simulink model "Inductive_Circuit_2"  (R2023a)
settings: Solver=VariableStepAuto  StartTime=0.0  StopTime=10.0  RelTol=1e-3
libraries: fl_lib x9

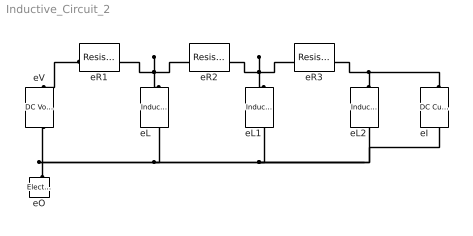
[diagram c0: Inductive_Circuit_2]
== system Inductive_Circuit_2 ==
  eI : fl_lib/Electrical/Electrical Sources/DC Current Source  i0=1 A
  eL : fl_lib/Electrical/Electrical Elements/Inductor  l=1e-6 H  r=0 Ohm  g=1e-9 1/Ohm  i_specify=off  i_priority=None  i=0 A  i_nominal_specify=off  i_nominal_unit=A  i_nominal_value=1  v_specify=off  v_priority=None  v=0 V  v_nominal_specify=off  v_nominal_unit=V  v_nominal_value=1  i_L_specify=off  i_L_priority=High  i_L=0 A  i_L_nominal_specify=off  i_L_nominal_unit=A  i_L_nominal_value=1
  eL1 : fl_lib/Electrical/Electrical Elements/Inductor  l=1e-6 H  r=0 Ohm  g=1e-9 1/Ohm  i_specify=off  i_priority=None  i=0 A  i_nominal_specify=off  i_nominal_unit=A  i_nominal_value=1  v_specify=off  v_priority=None  v=0 V  v_nominal_specify=off  v_nominal_unit=V  v_nominal_value=1  i_L_specify=off  i_L_priority=High  i_L=0 A  i_L_nominal_specify=off  i_L_nominal_unit=A  i_L_nominal_value=1
  eL2 : fl_lib/Electrical/Electrical Elements/Inductor  l=1e-6 H  r=0 Ohm  g=1e-9 1/Ohm  i_specify=off  i_priority=None  i=0 A  i_nominal_specify=off  i_nominal_unit=A  i_nominal_value=1  v_specify=off  v_priority=None  v=0 V  v_nominal_specify=off  v_nominal_unit=V  v_nominal_value=1  i_L_specify=off  i_L_priority=High  i_L=0 A  i_L_nominal_specify=off  i_L_nominal_unit=A  i_L_nominal_value=1
  eO : fl_lib/Electrical/Electrical Elements/Electrical Reference
  eR1 : fl_lib/Electrical/Electrical Elements/Resistor  R=1 Ohm  i_specify=off  i_priority=None  i=0 A  i_nominal_specify=off  i_nominal_unit=A  i_nominal_value=1  v_specify=off  v_priority=None  v=0 V  v_nominal_specify=off  v_nominal_unit=V  v_nominal_value=1
  eR2 : fl_lib/Electrical/Electrical Elements/Resistor  R=1 Ohm  i_specify=off  i_priority=None  i=0 A  i_nominal_specify=off  i_nominal_unit=A  i_nominal_value=1  v_specify=off  v_priority=None  v=0 V  v_nominal_specify=off  v_nominal_unit=V  v_nominal_value=1
  eR3 : fl_lib/Electrical/Electrical Elements/Resistor  R=1 Ohm  i_specify=off  i_priority=None  i=0 A  i_nominal_specify=off  i_nominal_unit=A  i_nominal_value=1  v_specify=off  v_priority=None  v=0 V  v_nominal_specify=off  v_nominal_unit=V  v_nominal_value=1
  eV : fl_lib/Electrical/Electrical Sources/DC Voltage Source  v0=1 V
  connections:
  eO/LConn1 -- eL/RConn1 -- eL1/RConn1 -- eL2/RConn1 -- eI/RConn1 -- eV/RConn1
  eR1/LConn1 -- eV/LConn1
  eL/LConn1 -- eR2/LConn1 -- eR1/RConn1
  eL1/LConn1 -- eR3/LConn1 -- eR2/RConn1
  eI/LConn1 -- eR3/RConn1 -- eL2/LConn1
